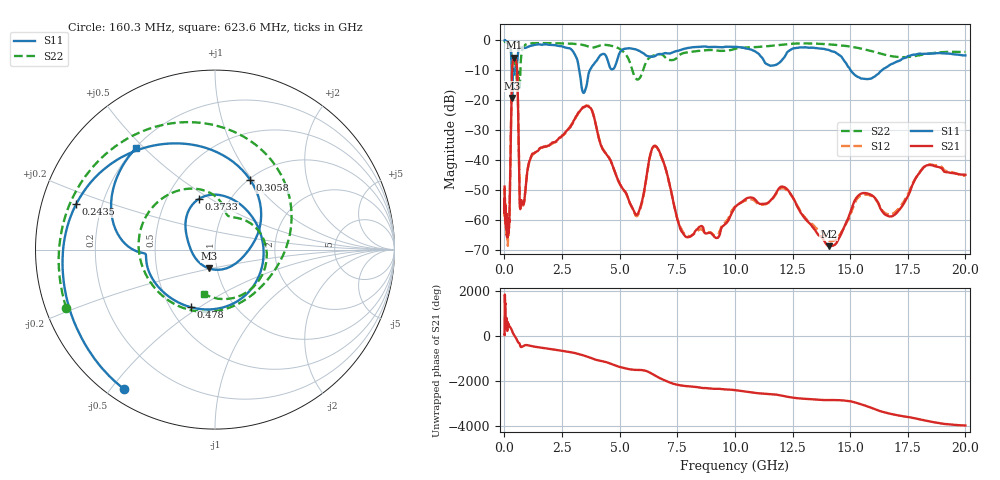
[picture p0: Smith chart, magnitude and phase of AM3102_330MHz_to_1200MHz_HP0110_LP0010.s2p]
! Date/Time: Tue, Sep 11, 2018 5:14 PM
! Network Analyzer: Agilent Technologies E8362B Rev: A.07.50.63
! Sweep from 0.010 to 20.000 GHz, 1601 Points, Sweep Type: LOG
! Power Supply: 4.949 V, 0.001 A
# Hz S DB R 50
!freq MagS11 AngS11 MagS21 AngS21 MagS12 AngS12 MagS22 AngS22
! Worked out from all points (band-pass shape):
!   1601 points, 10 MHz to 20 GHz, reference 50 ohm
!   highest |S21| = -5.78 dB at 426.5 MHz (marker M1); lowest = -68.6 dB at 14.07 GHz (marker M2)
!   |S21| within 3 dB of the highest: 342.3 MHz to 542.6 MHz (200.3 MHz wide, 45.3 % of centre)
!   lowest |S11| = -19.1 dB at 337.9 MHz (marker M3), VSWR 1.25, Z = 45.7 - j9.71 ohm
!   |S11| at or under -10 dB: 315 MHz to 455.8 MHz (140.8 MHz wide, 36.5 % of centre); 3.25 GHz to 3.702 GHz (452.4 MHz wide, 13 % of centre); 15.03 GHz to 16.37 GHz (1.344 GHz wide, 8.56 % of centre)
!   |S22| runs from -16.2 to -0.2 dB; largest |S21 - S12| = 0.0072
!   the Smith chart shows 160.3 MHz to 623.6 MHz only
!   S11 on the Smith chart (normalised r, x): 160.3 MHz: 0.05, -0.54; 243.5 MHz: 0.11, +0.16; 305.8 MHz: 1.02, +0.98; 373.3 MHz: 0.72, +0.45; 478 MHz: 0.63, -0.46; 623.6 MHz: 0.20, +0.47
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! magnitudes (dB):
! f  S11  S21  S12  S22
! 10 MHz  0.0  -48.7  -50.1  -0.2
! 35.55 MHz  0.0  -57.7  -57.2  -0.4
! 126.4 MHz  -0.4  -63.4  -63.2  -0.8
! 160.3 MHz  -0.6  -61.5  -64.4  -1.0
! 243.5 MHz  -1.8  -48.3  -48.4  -1.9
! 305.8 MHz  -7.2  -18.7  -18.7  -4.8
! 337.9 MHz  -19.1  -9.4  -9.5  -8.8
! 373.3 MHz  -10.6  -6.6  -6.7  -9.3
! 426.5 MHz  -11.3  -5.8  -5.8  -7.6
! 447.2 MHz  -10.4  -5.9  -5.9  -7.4
! 478 MHz  -9.2  -6.1  -6.2  -7.8
! 556.4 MHz  -7.3  -10.8  -11.0  -13.7
! 623.6 MHz  -2.9  -35.2  -35.3  -11.9
! 692.3 MHz  -2.4  -56.1  -56.4  -10.5
! 1.59 GHz  -1.4  -35.7  -35.8  -0.9
! 3.651 GHz  -11.1  -22.0  -21.8  -2.0
! 5.652 GHz  -2.9  -57.5  -57.7  -12.1
! 6.58 GHz  -5.0  -35.3  -35.5  -4.8
! 7.882 GHz  -2.6  -65.5  -65.0  -4.0
! 12.09 GHz  -6.1  -48.8  -49.3  -1.3
! 14.07 GHz  -3.2  -68.6  -66.7  -1.3
! 20 GHz  -5.0  -44.8  -45.1  -3.8
